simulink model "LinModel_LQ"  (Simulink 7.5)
settings: Solver=ode45  StartTime=0.0  StopTime=10.0  RelTol=1e-3
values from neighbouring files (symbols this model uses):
  dX0 = [0 0 0.55 0]'    [Exercises05.m]
  K = lqr(A,B,C'*Q*C,R)    [Exercises05.m]
undefined symbols (not defined in the file or in its folder): A, B, C

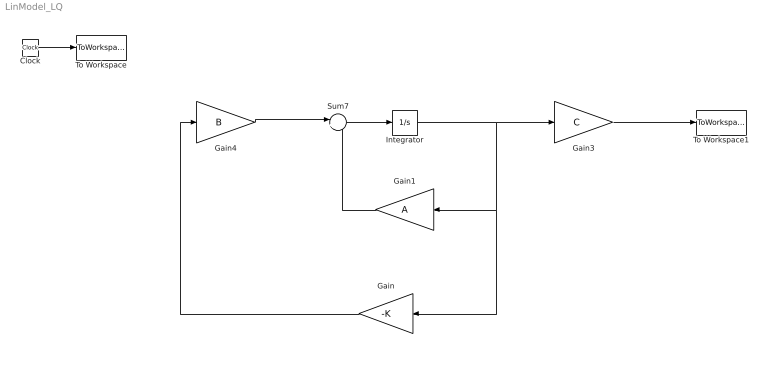
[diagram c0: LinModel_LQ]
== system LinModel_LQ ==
  Clock : Clock
  Gain : Gain  Gain=-K  Multiplication=Matrix(K*u)  ParameterDataType=fixdt(1, 16)  ParameterScaling=2^0  OutDataType=fixdt(1, 16)  OutScaling=2^0
  Gain1 : Gain  Gain=A  Multiplication=Matrix(K*u)  ParameterDataType=sfix(16)  ParameterScaling=2^0  OutDataType=sfix(16)  OutScaling=2^0
  Gain3 : Gain  Gain=C  Multiplication=Matrix(K*u)  ParameterDataType=sfix(16)  ParameterScaling=2^0  OutDataType=sfix(16)  OutScaling=2^0
  Gain4 : Gain  Gain=B  Multiplication=Matrix(K*u)  ParameterDataType=sfix(16)  ParameterScaling=2^0  OutDataType=sfix(16)  OutScaling=2^0
  Integrator : Integrator  InitialCondition=dX0
  Sum7 : Sum  Inputs=|++  OutDataType=sfix(16)  OutScaling=2^0
  To Workspace : ToWorkspace  VariableName=time  SampleTime=-1  SaveFormat=Array
  To Workspace1 : ToWorkspace  VariableName=dy  SampleTime=-1  SaveFormat=Array
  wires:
  Clock/1 -> To Workspace/1
  Integrator/1 -> Gain3/1, Gain1/1, Gain/1
  Sum7/1 -> Integrator/1
  Gain1/1 -> Sum7/2
  Gain4/1 -> Sum7/1
  Gain3/1 -> To Workspace1/1
  Gain/1 -> Gain4/1
